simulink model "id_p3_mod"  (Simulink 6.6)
settings: Solver=ode5  StartTime=0.0  StopTime=10.0  FixedStep=sample  RelTol=1e-3
undefined symbols (not defined in the file or in its folder): noise, sample, step_mag

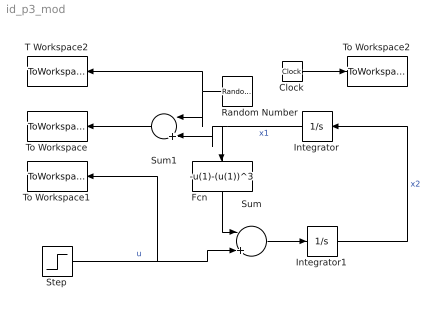
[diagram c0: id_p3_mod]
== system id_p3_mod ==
  Clock : Clock
  Fcn : Fcn  Orientation=down  Expr=-u(1)-(u(1))^3
  Integrator : Integrator  Orientation=left
  Integrator1 : Integrator
  Random Number : RandomNumber  Orientation=left  Variance=noise  SampleTime=0
  Step : Step  After=step_mag  SampleTime=0
  Sum : Sum  Inputs=|++
  Sum1 : Sum  Orientation=left  Inputs=|++
  T Workspace2 : ToWorkspace  VariableName=Noise  SampleTime=-1  SaveFormat=Array
  To Workspace : ToWorkspace  VariableName=x1  SampleTime=sample  SaveFormat=Array
  To Workspace1 : ToWorkspace  VariableName=u  SampleTime=sample  SaveFormat=Array
  To Workspace2 : ToWorkspace  VariableName=t  SampleTime=sample  SaveFormat=Array
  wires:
  Sum1/1 -> To Workspace/1
  Random Number/1 -> T Workspace2/1, Sum1/1
  Step/1 -> Sum/2, To Workspace1/1  "u"
  Fcn/1 -> Sum/1
  Sum/1 -> Integrator1/1
  Integrator/1 -> Fcn/1, Sum1/2  "x1"
  Integrator1/1 -> Integrator/1  "x2"
  Clock/1 -> To Workspace2/1
